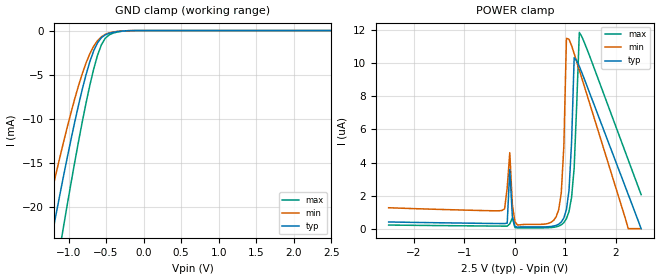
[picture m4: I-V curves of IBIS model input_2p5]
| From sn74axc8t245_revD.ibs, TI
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|   input_2p5 Model
[Model]   input_2p5
Model_type   Input
Vinl = 0.75
Vinh = 1.75
|   typ   min   max
C_comp   1.816pF   1.803pF   1.864pF
| Where Nom  PVT is Nominal Process, 2.5V, 27C
|   Fast PVT is Strong Process,  2.75V, -40C
|   Slow PVT is Weak Process,   2.25, 125C
[Voltage Range]   2.5   2.25   2.75
|Junction Temperature
[Temperature Range]   27   150   -40
[Power Clamp Reference]   2.5   2.25   2.75
[GND Clamp Reference]   0   0   0
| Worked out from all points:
|   GND clamp passes 1 mA (typ) near -0.58 V on its own axis
[GND Clamp]
|Voltage   I(typ)   I(min)   I(max)
-2.5V     -85.92mA   -72.48mA   -101.3mA
-1.378V   -30.54mA   -24.33mA   -38.61mA
-1.327V   -28.17mA   -22.33mA   -35.87mA
-1.225V   -23.5mA    -18.43mA   -30.45mA
-1.174V   -21.22mA   -16.53mA   -27.78mA
-1.072V   -16.75mA   -12.86mA   -22.53mA
-868mV    -8.5mA     -6.29mA    -12.65mA
-715mV    -3.502mA   -2.603mA   -6.167mA
-613mV    -1.378mA   -1.131mA   -2.784mA
-511mV    -483.8uA   -430.3uA   -873.9uA
-205mV    -15.33uA   -14.93uA   -16.6uA
2.5V      0A         0A         0A
[POWER_clamp]
|Voltage   I(typ)   I(min)   I(max)
-2.5V     405.1nA    1.265uA    219.4nA
-254mV    308nA      1.102uA    153.5nA
-152mV    332.4nA    2.482uA    152.6nA
-101mV    3.587uA    4.599uA    287.5nA
1mV       136.9nA    414.1nA    63.89nA
766mV     156.4nA    497.3nA    83.48nA
919mV     401.6nA    2.172uA    232.7nA
1.021V    1.162uA    11.52uA    603.1nA
1.123V    5.246uA    11.07uA    1.901uA
1.174V    10.34uA    10.59uA    3.674uA
1.276V    9.816uA    9.587uA    11.87uA
2.5V      0A         0A         2.058uA
